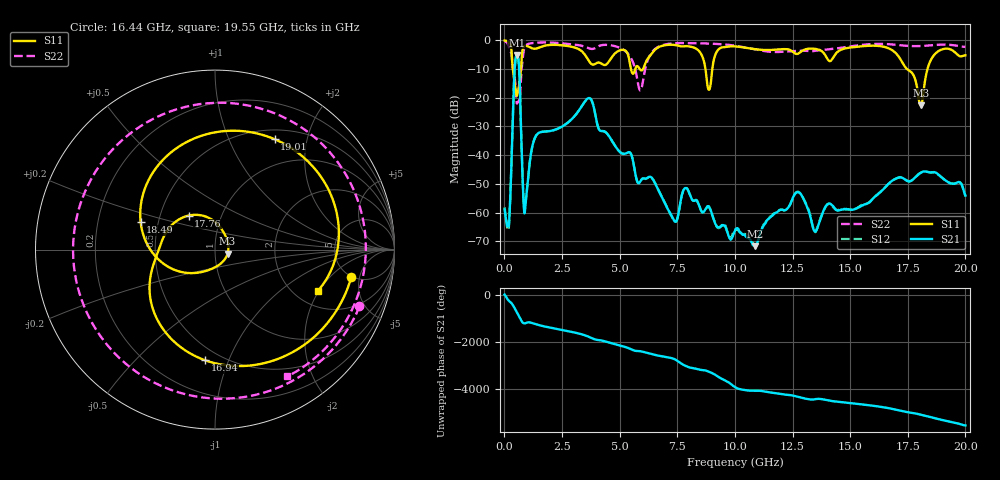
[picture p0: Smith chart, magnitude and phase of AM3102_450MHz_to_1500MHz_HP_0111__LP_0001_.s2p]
!Agilent Technologies,E8364B,MY43040894,A.07.50.67
!Agilent E8364B: A.07.50.67
!Date: Thursday, January 11, 2018 05:51:06
!Correction: S11(Full 2 Port(1,2))
!S21(Full 2 Port(1,2))
!S12(Full 2 Port(1,2))
!S22(Full 2 Port(1,2))
!S2P File: Measurements: S11, S21, S12, S22:
# Hz S  dB  R 50
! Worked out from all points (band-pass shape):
!   1601 points, 10 MHz to 20 GHz, reference 50 ohm
!   highest |S21| = -5.13 dB at 534.7 MHz (marker M1); lowest = -71.7 dB at 10.88 GHz (marker M2)
!   |S21| within 3 dB of the highest: 464.3 MHz to 625.5 MHz (161.2 MHz wide, 29.6 % of centre)
!   lowest |S11| = -22.7 dB at 18.06 GHz (marker M3), VSWR 1.16, Z = 57.5 - j2.58 ohm
!   |S11| at or under -10 dB: 367.1 MHz to 721.2 MHz (354.1 MHz wide, 65.1 % of centre); 8.724 GHz to 9.02 GHz (295.6 MHz wide, 3.33 % of centre); 17.46 GHz to 18.36 GHz (890.8 MHz wide, 4.97 % of centre)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
!   |S22| runs from -22.0 to -0.3 dB; largest |S21 - S12| = 0.004
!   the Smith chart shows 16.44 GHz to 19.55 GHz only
!   S11 on the Smith chart (normalised r, x): 16.44 GHz: 4.90, -3.77; 16.94 GHz: 0.41, -0.83; 17.76 GHz: 0.70, +0.28; 18.49 GHz: 0.40, +0.15; 19.01 GHz: 0.62, +1.49; 19.55 GHz: 2.62, -1.95
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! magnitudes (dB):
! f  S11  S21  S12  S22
! 10 MHz  -0.1  -58.8  -58.1  -0.3
! 197.4 MHz  -0.7  -64.0  -64.6  -2.5
! 534.7 MHz  -19.4  -5.1  -5.1  -21.8
! 897.1 MHz  -2.0  -58.9  -58.3  -2.2
! 1.384 GHz  -2.9  -33.1  -33.1  -0.8
! 3.346 GHz  -3.7  -23.1  -23.1  -1.9
! 5.895 GHz  -10.2  -49.2  -49.1  -17.5
! 6.682 GHz  -2.4  -52.2  -52.1  -2.3
! 8.881 GHz  -17.2  -58.0  -58.0  -1.1
! 10.01 GHz  -2.1  -66.3  -66.1  -1.9
! 10.88 GHz  -3.1  -71.7  -71.3  -3.2
! 12.69 GHz  -4.8  -52.9  -52.8  -3.7
! 13.34 GHz  -2.9  -63.5  -63.7  -3.8
! 16.44 GHz  -2.2  -51.9  -51.8  -1.3
! 16.68 GHz  -2.8  -49.9  -49.9  -1.4
! 16.94 GHz  -4.2  -48.3  -48.3  -1.5
! 17.76 GHz  -12.4  -48.2  -48.1  -2.0
! 18.06 GHz  -22.7  -46.1  -46.1  -2.0
! 18.49 GHz  -7.1  -46.0  -46.0  -1.8
! 19.01 GHz  -3.1  -48.0  -48.1  -1.5
! 19.55 GHz  -4.2  -49.9  -49.8  -1.8
! 20 GHz  -5.2  -54.0  -54.2  -2.3
